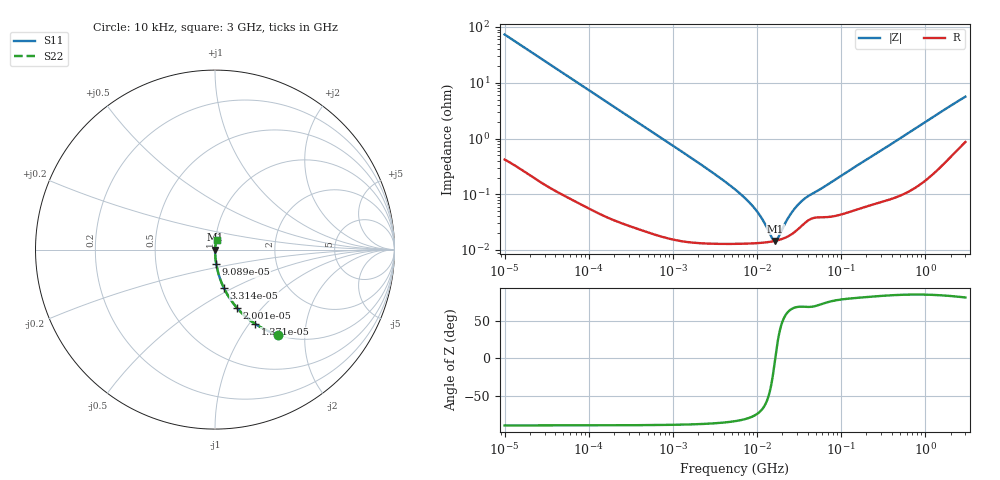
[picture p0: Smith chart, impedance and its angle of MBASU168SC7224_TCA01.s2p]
! MBASU168SC7224_TCA01  S-PARAMETER MODEL  ( Standard Model )
! Model Generated by TAIYO YUDEN Corporation (http://www.ty-top.com)
! Version 1.0
! TAIYO YUDEN Control No. 220601
! Copyright(c) 2016 TAIYO YUDEN CO.,LTD. All Rights Reserved.
! Product Description (link to TY-COMPAS)
! https://ds.yuden.co.jp/TYCOMPAS/or/detail?pn=MBASU168SC7224KTCA01&u=M
! Products Name : Multilayer Ceramic Capacitors
! Characteristics :
!  Capacitance : 0.22 [uF] , Rated Voltage : 50 [V] , TCC : X7S
!  Case Size : 1.6 x 0.8 / 0.063 x 0.031 [mm/inch] , Thickness : 0.8 / 0.031 [mm/inch]
!  (Conditions: Temperature = 25 [degC] , DC Bias Voltage = 0 [V])
! External Node Assignments :
!  1  o---| |---o  2
! GND o---------o GND
! Frequency Range : 10kHz  -  3GHz  [ 401 STEP ]
# MHZ S RI R 50
! Freq[MHz].  S11 Real  S11 Imag  S21 Real  S21 Imag  S12 Real  S12 Imag  S22 Real  S22 Imag
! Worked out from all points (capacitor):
!   401 points, 10 kHz to 3 GHz, reference 50 ohm
!   read as one part in series: C = 216 nF near 10.65 kHz
!   lowest |Z| = 14.6 mohm at 16.51 MHz (marker M1)
!   series resonance near 16.48 MHz, so ESL is about 430 pH
!   S11 on the Smith chart (normalised r, x): 10 kHz: 1.01, -1.47; 13.71 kHz: 1.01, -1.07; 20.01 kHz: 1.00, -0.74; 33.14 kHz: 1.00, -0.45; 90.89 kHz: 1.00, -0.16; 3 GHz: 1.02, +0.11
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0.01  0.3518 -0.4747  0.6482 0.4747  0.6482 0.4747  0.3518 -0.4747
0.013707  0.2253 -0.4149  0.7747 0.4149  0.7747 0.4149  0.2253 -0.4149
0.02001  0.1211 -0.3233  0.8789 0.3233  0.8789 0.3233  0.1211 -0.3233
0.033138  0.0485 -0.2118  0.9515 0.2118  0.9515 0.2118  0.0485 -0.2118
0.082683  0.0086 -0.0888  0.9914 0.0888  0.9914 0.0888  0.0086 -0.0888
0.090886  0.0072 -0.0809  0.9928 0.0809  0.9928 0.0809  0.0072 -0.0809
0.212913  0.00155 -0.0349  0.9985 0.0349  0.9985 0.0349  0.00155 -0.0349
0.683653  0.000298 -0.0109  0.9997 0.0109  0.9997 0.0109  0.000298 -0.0109
2.652321  0.000138 -0.00275  0.9999 0.00275  0.9999 0.00275  0.000138 -0.00275
5.477226  0.00013 -0.00122  0.9999 0.00122  0.9999 0.00122  0.00013 -0.00122
7.507384  0.000131 -0.000793  0.9999 0.000793  0.9999 0.000793  0.000131 -0.000793
9.6612  0.000133 -0.000511  0.9999 0.000511  0.9999 0.000511  0.000133 -0.000511
11.67315  0.000135 -0.000322  0.9999 0.000322  0.9999 0.000322  0.000135 -0.000322
15.02209  0.000142 -8.53e-05  0.9999 8.53e-05  0.9999 8.53e-05  0.000142 -8.53e-05
16.51234  0.000146 1.57e-06  0.9999 -1.57e-06  0.9999 -1.57e-06  0.000146 1.57e-06
17.5871  0.000149 5.96e-05  0.9999 -5.96e-05  0.9999 -5.96e-05  0.000149 5.96e-05
22.63272  0.000172 0.000298  0.9998 -0.000298  0.9998 -0.000298  0.000172 0.000298
28.22191  0.000212 0.000518  0.9998 -0.000518  0.9998 -0.000518  0.000212 0.000518
35.19136  0.000286 0.000737  0.9997 -0.000737  0.9997 -0.000737  0.000286 0.000737
45.28751  0.00037 0.000953  0.9996 -0.000953  0.9996 -0.000953  0.00037 0.000953
374.4521  0.000857 0.00752  0.9991 -0.00752  0.9991 -0.00752  0.000857 0.00752
3000  0.0116 0.0546  0.9884 -0.0546  0.9884 -0.0546  0.0116 0.0546
